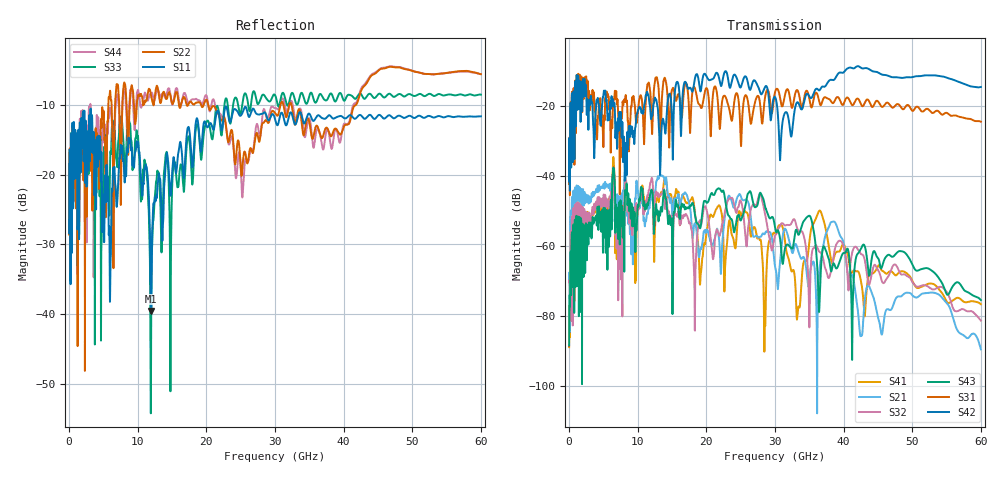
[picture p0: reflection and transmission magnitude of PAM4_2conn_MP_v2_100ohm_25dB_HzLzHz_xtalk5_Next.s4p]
! Info: Touchstone file created by Circ.  Input file=FAB50GbE_2conn_Midplane_Examax_Topo2_v2_100ohm_25dB_HzLzHz.circ
# Hz S RI R 50
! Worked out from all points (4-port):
!   6000 points, 10 MHz to 60 GHz, reference 50 ohm
!   strongest paths, dB at 10 MHz, 15.01 GHz, 30.01 GHz, 45.01 GHz, 60 GHz:
!     S42: -41.6, -24.7, -17.5, -10.5, -14.7
!     S31: -42.3, -15.4, -16.1, -18.8, -24.6
!     S43: -88.5, -56.7, -54.8, -63.5, -75.5
!     S32: -70.2, -54.2, -57.2, -66.9, -81.4
!     S21: -69.8, -50.1, -65.9, -80.4, -89.6
!     S41: -89.0, -48.5, -56.5, -65.8, -76.7
!   lowest |S11| = -39.6 dB at 11.98 GHz (marker M1), VSWR 1.02, Z = 51 + j0.162 ohm
!   |S11| at or under -10 dB: start of sweep to end of sweep
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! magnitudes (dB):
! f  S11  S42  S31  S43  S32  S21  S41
! 10 MHz  -28.4  -41.6  -42.3  -88.5  -70.2  -69.8  -89.0
! 1.35 GHz  -13.6  -11.9  -11.0  -56.0  -49.8  -43.0  -51.2
! 11.98 GHz  -39.6  -23.6  -22.1  -44.0  -41.0  -45.9  -45.0
! 18.3 GHz  -14.4  -12.7  -14.8  -50.7  -76.4  -53.6  -50.0
! 27.82 GHz  -11.3  -16.0  -19.3  -44.9  -45.2  -57.4  -58.4
! 36.43 GHz  -11.5  -15.6  -18.7  -78.9  -61.6  -68.2  -50.1
! 60 GHz  -11.6  -14.7  -24.6  -75.5  -81.4  -89.6  -76.7
